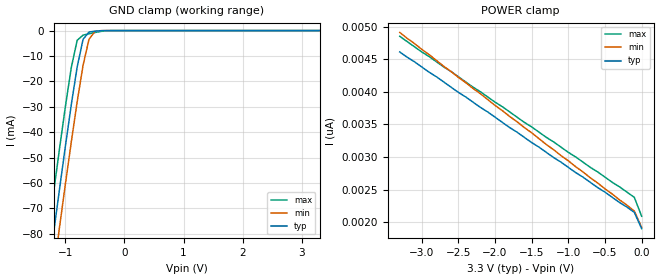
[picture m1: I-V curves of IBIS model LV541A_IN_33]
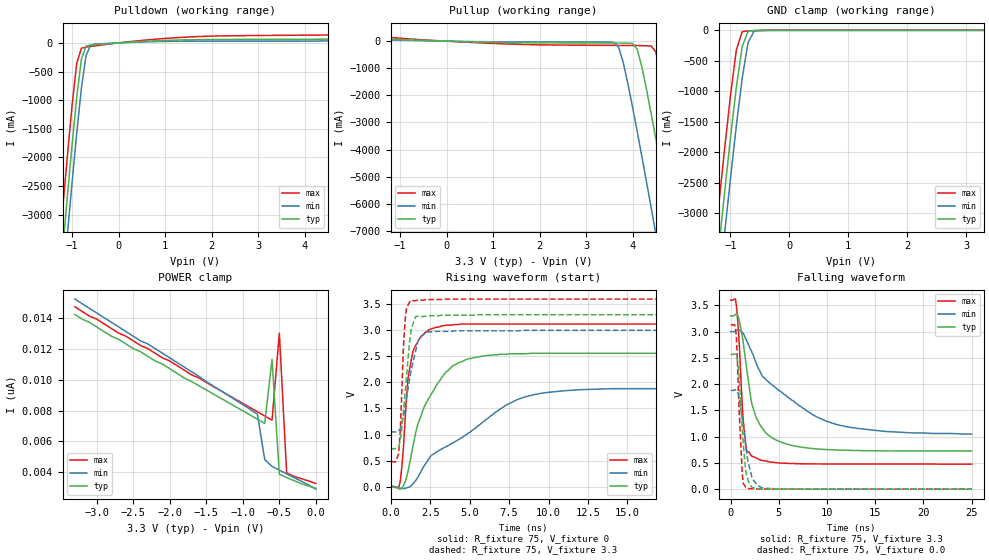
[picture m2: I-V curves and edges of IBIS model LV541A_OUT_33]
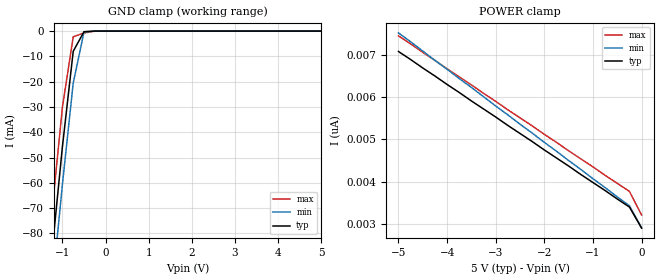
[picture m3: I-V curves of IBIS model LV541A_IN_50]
| TEXAS INSTRUMENTS INCORPORATED
| Standard Linear and Logic Group
| IBIS Model of SN74LV541A
| OCTAL BUFFER/DRIVER WITH 3-STATE OUTPUTS
| SOIC 20-pin (DW), SOP 20-pin (NS), SSOP 20-pin (DB), TSSOP 20-pin (PW)
| and TVSOP 20-pin (DGV) Package
[IBIS Ver]   3.2
[Comment Char]  |_char
[File Name]   lv541a.ibs
[File Rev]   2.0 H_die
[Date]   May 29, 2000
[Source]   Data created from HSPICE simulations at TI-SLL.
[Notes]   The following is an IBIS list for the LV541A.
|   Please contact sllibis@ti.com with questions and
|   comments concerning SLL IBIS models.
|   The warning about non-monotonic V-I curves might be reported,
|   but it is nano ampere region and negligible.
[Disclaimer] Property of Texas Instruments Incorporated.  Unauthorized
   reproduction and/or distribution is strictly prohibited.
   This product is protected under copyright law.
   Created 2000, (C) Copyright 2000, Texas Instruments Inc.,
   All Rights Reserved.
   UNLESS THERE IS A SIGNED, WRITTEN AGREEMENT TO THE
   CONTRARY, TEXAS INSTRUMENTS () IS PROVIDING THE IBIS
   MODELS  AND WITHOUT ANY WARRANTY, EXPRESSED OR
   IMPLIED.  TI assumes no liability for:
   1) the accuracy of the IBIS models provided to your
   company;
   2) the proper functioning of these IBIS Models in your
   design or for any resulting applications; or
   3) infringement of patents, copyrights or intellectual
   property rights resulting from your use of these IBIS
   models.
   TI provides IBIS Models as a service to our customers.
   You and your company shall not distribute, sell or give
   these models to anyone else without prior written
   permission from TI.
   TI reserves the right to make changes to our products or
   to discontinue any semiconductor product or service
   without notice, and advises our customers to obtain the
   latest version of relevant information to verify, before
   placing orders, that the information being relied on is
   current.
   Please be aware that your receipt and use of the IBIS
   information provided shall serve as acceptance of these
   terms and conditions.  If you do not accept these terms,
   you should return or destroy the IBIS models and any
   other accompanying information immediately.
|   Component LV541A_DW
[Component]   LV541A_DW
[Manufacturer]  Texas Instruments, Inc.
[Package]
|   typ   min   max
R_pkg   0.038   0.033   0.045
L_pkg   5.012nH   4.110nH   6.349nH
C_pkg   0.717pF   0.530pF   0.868pF
[Pin]   signal_name   model_name   R_pin   L_pin   C_pin
1   OE1_NOT   LV541A_IN   0.042   6.336nH   0.865pF
2   A1   LV541A_IN   0.043   5.542nH   0.867pF
3   A2   LV541A_IN   0.034   4.714nH   0.732pF
4   A3   LV541A_IN   0.034   4.377nH   0.591pF
5   A4   LV541A_IN   0.036   4.130nH   0.533pF
6   A5   LV541A_IN   0.035   4.111nH   0.530pF
7   A6   LV541A_IN   0.034   4.284nH   0.583pF
8   A7   LV541A_IN   0.034   4.634nH   0.726pF
9   A8   LV541A_IN   0.040   5.518nH   0.865pF
10   GND   GND   0.043   6.349nH   0.866pF
11   Y8   LV541A_OUT   0.041   6.281nH   0.861pF
12   Y7   LV541A_OUT   0.045   5.561nH   0.868pF
13   Y6   LV541A_OUT   0.033   4.778nH   0.742pF
14   Y5   LV541A_OUT   0.035   4.414nH   0.596pF
15   Y4   LV541A_OUT   0.035   4.110nH   0.533pF
16   Y3   LV541A_OUT   0.036   4.130nH   0.533pF
17   Y2   LV541A_OUT   0.034   4.377nH   0.591pF
18   Y1   LV541A_OUT   0.034   4.714nH   0.731pF
19   OE2_NOT   LV541A_IN   0.043   5.569nH   0.868pF
20   VCC   POWER   0.042   6.308nH   0.864pF
|   Component LV541A_NS
[Component]   LV541A_NS
[Manufacturer]  Texas Instruments, Inc.
[Package]
|   typ   min   max
R_pkg   0.044   0.029   0.058
L_pkg   3.666nH   2.317nH   5.115nH
C_pkg   0.548pF   0.316pF   0.725pF
[Pin]   signal_name   model_name   R_pin   L_pin   C_pin
1   OE1_NOT   LV541A_IN   0.058   5.115nH   0.725pF
2   A1   LV541A_IN   0.053   4.591nH   0.724pF
3   A2   LV541A_IN   0.049   3.754nH   0.572pF
4   A3   LV541A_IN   0.029   2.549nH   0.388pF
5   A4   LV541A_IN   0.031   2.317nH   0.316pF
6   A5   LV541A_IN   0.031   2.317nH   0.316pF
7   A6   LV541A_IN   0.029   2.556nH   0.399pF
8   A7   LV541A_IN   0.049   3.754nH   0.579pF
9   A8   LV541A_IN   0.053   4.591nH   0.724pF
10   GND   GND   0.058   5.115nH   0.725pF
11   Y8   LV541A_OUT   0.058   5.115nH   0.725pF
12   Y7   LV541A_OUT   0.053   4.591nH   0.724pF
13   Y6   LV541A_OUT   0.049   3.754nH   0.579pF
14   Y5   LV541A_OUT   0.029   2.557nH   0.399pF
15   Y4   LV541A_OUT   0.031   2.317nH   0.316pF
16   Y3   LV541A_OUT   0.031   2.317nH   0.316pF
17   Y2   LV541A_OUT   0.029   2.557nH   0.399pF
18   Y1   LV541A_OUT   0.049   3.754nH   0.579pF
19   OE2_NOT   LV541A_IN   0.053   4.591nH   0.724pF
20   VCC   POWER   0.058   5.115nH   0.725pF
|   Component LV541A_DB
[Component]   LV541A_DB
[Manufacturer]  Texas Instruments, Inc.
[Package]
|   typ   min   max
R_pkg   0.040   0.035   0.051
L_pkg   3.495nH   3.035nH   4.314nH
C_pkg   0.420pF   0.346pF   0.502pF
[Pin]   signal_name   model_name   R_pin   L_pin   C_pin
1   OE1_NOT   LV541A_IN   0.049   4.310nH   0.502pF
2   A1   LV541A_IN   0.048   3.903nH   0.487pF
3   A2   LV541A_IN   0.035   3.189nH   0.396pF
4   A3   LV541A_IN   0.035   3.036nH   0.347pF
5   A4   LV541A_IN   0.035   3.035nH   0.367pF
6   A5   LV541A_IN   0.035   3.035nH   0.367pF
7   A6   LV541A_IN   0.035   3.036nH   0.347pF
8   A7   LV541A_IN   0.035   3.189nH   0.397pF
9   A8   LV541A_IN   0.047   3.899nH   0.488pF
10   GND   GND   0.051   4.314nH   0.500pF
11   Y8   LV541A_OUT   0.051   4.314nH   0.500pF
12   Y7   LV541A_OUT   0.047   3.899nH   0.488pF
13   Y6   LV541A_OUT   0.035   3.189nH   0.397pF
14   Y5   LV541A_OUT   0.035   3.036nH   0.346pF
15   Y4   LV541A_OUT   0.035   3.035nH   0.367pF
16   Y3   LV541A_OUT   0.035   3.035nH   0.367pF
17   Y2   LV541A_OUT   0.035   3.036nH   0.346pF
18   Y1   LV541A_OUT   0.035   3.189nH   0.397pF
19   OE2_NOT   LV541A_IN   0.047   3.899nH   0.488pF
20   VCC   POWER   0.051   4.314nH   0.502pF
|   Component LV541A_PW
[Component]   LV541A_PW
[Manufacturer]  Texas Instruments, Inc.
[Package]
|   typ   min   max
R_pkg   0.035   0.024   0.047
L_pkg   2.399nH   1.710nH   3.250nH
C_pkg   0.284pF   0.166pF   0.418pF
[Pin]   signal_name   model_name   R_pin   L_pin   C_pin
1   OE1_NOT   LV541A_IN   0.041   3.102nH   0.410pF
2   A1   LV541A_IN   0.040   2.777nH   0.363pF
3   A2   LV541A_IN   0.029   2.194nH   0.260pF
4   A3   LV541A_IN   0.025   1.710nH   0.166pF
5   A4   LV541A_IN   0.025   1.740nH   0.191pF
6   A5   LV541A_IN   0.024   1.763nH   0.193pF
7   A6   LV541A_IN   0.024   1.817nH   0.174pF
8   A7   LV541A_IN   0.028   2.256nH   0.265pF
9   A8   LV541A_IN   0.045   2.887nH   0.368pF
10   GND   GND   0.047   3.250nH   0.417pF
11   Y8   LV541A_OUT   0.046   3.244nH   0.418pF
12   Y7   LV541A_OUT   0.046   2.961nH   0.375pF
13   Y6   LV541A_OUT   0.033   2.334nH   0.268pF
14   Y5   LV541A_OUT   0.029   1.915nH   0.179pF
15   Y4   LV541A_OUT   0.031   1.934nH   0.203pF
16   Y3   LV541A_OUT   0.032   1.917nH   0.201pF
17   Y2   LV541A_OUT   0.030   1.833nH   0.173pF
18   Y1   LV541A_OUT   0.036   2.324nH   0.268pF
19   OE2_NOT   LV541A_IN   0.042   2.869nH   0.372pF
20   VCC   POWER   0.042   3.160nH   0.414pF
|   Component LV541A_DGV
[Component]   LV541A_DGV
[Manufacturer]  Texas Instruments, Inc.
[Package]
|   typ   min   max
R_pkg   0.044   0.038   0.048
L_pkg   2.561nH   2.236nH   2.961nH
C_pkg   0.342pF   0.264pF   0.446pF
[Pin]   signal_name   model_name   R_pin   L_pin   C_pin
1   OE1_NOT   LV541A_IN   0.044   2.935nH   0.417pF
2   A1   LV541A_IN   0.042   2.869nH   0.446pF
3   A2   LV541A_IN   0.043   2.399nH   0.316pF
4   A3   LV541A_IN   0.044   2.236nH   0.265pF
5   A4   LV541A_IN   0.046   2.278nH   0.264pF
6   A5   LV541A_IN   0.045   2.274nH   0.264pF
7   A6   LV541A_IN   0.044   2.285nH   0.269pF
8   A7   LV541A_IN   0.043   2.452nH   0.320pF
9   A8   LV541A_IN   0.044   2.900nH   0.446pF
10   GND   GND   0.044   2.961nH   0.418pF
11   Y8   LV541A_OUT   0.045   2.954nH   0.418pF
12   Y7   LV541A_OUT   0.042   2.847nH   0.443pF
13   Y6   LV541A_OUT   0.045   2.453nH   0.319pF
14   Y5   LV541A_OUT   0.045   2.297nH   0.269pF
15   Y4   LV541A_OUT   0.048   2.334nH   0.268pF
16   Y3   LV541A_OUT   0.048   2.335nH   0.267pF
17   Y2   LV541A_OUT   0.046   2.299nH   0.268pF
18   Y1   LV541A_OUT   0.046   2.457nH   0.320pF
19   OE2_NOT   LV541A_IN   0.043   2.848nH   0.441pF
20   VCC   POWER   0.038   2.812nH   0.408pF
[Model Selector]   LV541A_IN
LV541A_IN_33   3.3-V Vcc Input Model
LV541A_IN_50   5.0-V Vcc Input Model
[Model Selector]   LV541A_OUT
LV541A_OUT_33   3.3-V Vcc Output Model
LV541A_OUT_50   5.0-V Vcc Output Model
| Models and submodels in the file (4): LV541A_IN_33 (Input), LV541A_OUT_33 (3-state), LV541A_IN_50 (Input), LV541A_OUT_50 (3-state)
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|   Model LV541A_IN_33
[Model]   LV541A_IN_33
Model_type  Input
Polarity   Inverting
Vinl = 0.99
Vinh = 2.31
| variable   typ   min   max
C_comp   1.33pf   1.00pf   1.66pf
[Temperature Range]   25   85   -40
[Voltage Range]   3.3   3.0   3.6
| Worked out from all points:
|   GND clamp passes 1 mA (typ) near -0.61 V on its own axis
[GND Clamp]
|   Voltage   I(typ)   I(min)   I(max)
-3.3V     -460mA     -475mA     -445mA
-1.3V     -97.5mA    -113mA     -81.5mA
-1.2V     -79.9mA    -95mA      -63.9mA
-1.1V     -62.6mA    -77.6mA    -46.7mA
-1V       -45.6mA    -60.5mA    -30mA
-900mV    -29.2mA    -43.9mA    -14.6mA
-800mV    -14.3mA    -28mA      -3.81mA
-700mV    -3.42mA    -13.6mA    -1.78mA
-600mV    -581uA     -3.4mA     -1.25mA
-500mV    -233uA     -353uA     -759uA
-400mV    -58.1uA    -21.9uA    -324uA
3.3V      1.9nA      2.34nA     1.69nA
[POWER Clamp]
|   Voltage   I(typ)   I(min)   I(max)
-3.3V     4.61nA     4.91nA     4.85nA
-3V       4.38nA     4.65nA     4.61nA
-100mV    2.15nA     2.17nA     2.38nA
0V        1.9nA      1.92nA     2.09nA
|   Model LV541A_OUT_33
[Model]   LV541A_OUT_33
Model_type  3-state
Polarity   Non-Inverting
Enable   Active-Low
Vinl = 0.99
Vinh = 2.31
Vmeas = 1.65v
Cref = 15pf
| variable   typ   min   max
C_comp   4.60pf   3.45pf   5.75pf
[Temperature Range]   25   85   -40
[Voltage Range]   3.3   3.0   3.6
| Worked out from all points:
|   slope of the pulldown table from 0 to 0.495 V, typ, clamps not added: 19.7 ohm
|   slope of the pullup table from 0 to 0.495 V, typ, clamps not added: 20.4 ohm
|   GND clamp passes 1 mA (typ) near -0.48 V on its own axis
|   rising waveform, R_fixture 75, V_fixture 0: 20-80 % time 1.89ns typ, 4.98ns min, 570ps max; typ from 0 V to 2.56 V
|   falling waveform, R_fixture 75, V_fixture 3.3: 20-80 % time 1.69ns typ, 6.13ns min, 606ps max; typ from 3.3 V to 0.726 V
|   rising waveform, R_fixture 75, V_fixture 3.3: 20-80 % time 456ps typ, 722ps min, 258ps max; typ from 0.726 V to 3.3 V
|   falling waveform, R_fixture 75, V_fixture 0.0: 20-80 % time 570ps typ, 928ps min, 429ps max; typ from 2.57 V to 0 V
[Pulldown]
|   Voltage   I(typ)   I(min)   I(max)
-3.3V     -24.1A     -24.7A     -23.5A
-1.3V     -4.54A     -5.2A      -3.83A
-1.2V     -3.6A      -4.26A     -2.88A
-1.1V     -2.67A     -3.34A     -1.97A
-1V       -1.78A     -2.44A     -1.09A
-900mV    -948mA     -1.58A     -358mA
-800mV    -288mA     -793mA     -92.6mA
-700mV    -55.7mA    -219mA     -74.5mA
-600mV    -37.6mA    -37.4mA    -63.2mA
0V        -3.42nA    -3.55nA    -3.6nA
1.6V      55.7mA     30.4mA     107mA
6.6V      122mA      69mA       228mA
[Pullup]
|   Voltage   I(typ)   I(min)   I(max)
-3.3V     223mA      124mA      415mA
600mV     -28.8mA    -16.4mA    -52.8mA
3.6V      -70.4mA    -45mA      -156mA
3.7V      -71mA      -222mA     -157mA
3.8V      -72.1mA    -794mA     -158mA
4.1V      -302mA     -3.34A     -163mA
4.4V      -2.68A     -6.15A     -177mA
4.5V      -3.6A      -7.11A     -395mA
4.8V      -6.45A     -10A       -2.89A
4.9V      -7.41A     -11A       -3.83A
5.2V      -10.3A     -13.9A     -6.71A
6.6V      -24.1A     -27.7A     -20.5A
[GND Clamp]
|   Voltage   I(typ)   I(min)   I(max)
-3.3V     -24.1A     -24.7A     -23.5A
-1.3V     -4.53A     -5.2A      -3.82A
-1.2V     -3.59A     -4.26A     -2.88A
-1.1V     -2.67A     -3.34A     -1.96A
-1V       -1.77A     -2.44A     -1.08A
-900mV    -938mA     -1.57A     -325mA
-800mV    -266mA     -785mA     -21.9mA
-700mV    -17.6mA    -203mA     -9.17mA
-600mV    -2.58mA    -15.3mA    -6.43mA
-400mV    -298uA     -33.8uA    -1.7mA
3.3V      2.97nA     3.67nA     2.84nA
[POWER Clamp]
|   Voltage   I(typ)   I(min)   I(max)
-3.3V     14.2nA     15.2nA     14.7nA
-2.5V     12nA       12.8nA     12.5nA
-2.4V     11.8nA     12.5nA     12.2nA
-2.3V     11.5nA     12.3nA     12nA
-1.7V     9.87nA     10.5nA     10.3nA
-1.6V     9.6nA      10.2nA     10.1nA
-800mV    7.44nA     7.76nA     7.92nA
-700mV    7.17nA     4.83nA     7.65nA
-600mV    11.3nA     4.39nA     7.38nA
-500mV    3.89nA     4.15nA     13nA
-400mV    3.67nA     3.91nA     3.98nA
0V        2.97nA     2.92nA     3.29nA
[Ramp]
| variable   typ   min   max
dV/dt_r   1.54E+00/1.89E-09   1.14E+00/5.03E-09   1.87E+00/5.53E-10
dV/dt_f   1.57E+00/1.70E-09   1.19E+00/6.17E-09   1.89E+00/5.89E-10
R_load = 75
[Rising Waveform]
R_fixture = 75
V_fixture = 0
|   Time   V(typ)   V(min)   V(max)
0s        0V         0V         0V
600ps     -49.1mV    -28.6mV    89.3mV
800ps     11.1mV     -38.5mV    712mV
1.1ns     292mV      -15mV      2.08V
1.4ns     756mV      52.7mV     2.59V
1.7ns     1.18V      168mV      2.77V
2.4ns     1.69V      524mV      3.01V
4.3ns     2.38V      903mV      3.11V
9ns       2.56V      1.76V      3.12V
25ns      2.56V      1.89V      3.12V
[Falling Waveform]
R_fixture = 75
V_fixture = 3.3
V_fixture_min = 3.0
V_fixture_max = 3.6
|   Time   V(typ)   V(min)   V(max)
0s        3.3V       3V         3.6V
500ps     3.33V      3.01V      3.62V
800ps     3.28V      3.03V      3.04V
1.3ns     2.8V       2.97V      1.32V
1.7ns     2.24V      2.81V      707mV
2.2ns     1.62V      2.61V      629mV
3ns       1.24V      2.26V      563mV
4.1ns     1V         2.01V      516mV
10ns      754mV      1.29V      479mV
25ns      726mV      1.05V      477mV
[Rising Waveform]
R_fixture = 75
V_fixture = 3.3
V_fixture_min = 3.0
V_fixture_max = 3.6
|   Time   V(typ)   V(min)   V(max)
0s        726mV      1.05V      477mV
500ps     766mV      1.06V      627mV
600ps     870mV      1.11V      1.03V
800ps     1.43V      1.34V      2.63V
900ps     1.76V      1.5V       3.14V
1ns       2.11V      1.69V      3.43V
1.3ns     3.01V      2.24V      3.58V
1.8ns     3.27V      2.84V      3.58V
2.3ns     3.28V      2.97V      3.59V
25ns      3.3V       3V         3.6V
[Falling Waveform]
R_fixture = 75
V_fixture = 0.0
|   Time   V(typ)   V(min)   V(max)
0s        2.57V      1.88V      3.13V
500ps     2.57V      1.89V      3.09V
600ps     2.54V      1.88V      2.86V
800ps     2.3V       1.8V       1.88V
1.2ns     1.15V      1.35V      315mV
1.5ns     459mV      919mV      52.1mV
1.7ns     240mV      625mV      14.2mV
2.3ns     30.8mV     187mV      5.9mV
3.3ns     8.02mV     23.2mV     2.94mV
25ns      72.5uV     112uV      75.9uV
|   Model LV541A_IN_50
[Model]   LV541A_IN_50
Model_type  Input
Polarity   Inverting
Vinl = 1.5
Vinh = 3.5
| variable   typ   min   max
C_comp   1.33pf   1.00pf   1.66pf
[Temperature Range]   25   85   -40
[Voltage Range]   5.0   4.5   5.5
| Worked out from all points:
|   GND clamp passes 1 mA (typ) near -0.52 V on its own axis
[GND Clamp]
|   Voltage   I(typ)   I(min)   I(max)
-5V       -773mA     -786mA     -758mA
-1.5V     -133mA     -148mA     -117mA
-1.25V    -88.7mA    -104mA     -72.7mA
-1V       -45.6mA    -60.5mA    -30mA
-750mV    -7.99mA    -20.5mA    -2.23mA
-500mV    -233uA     -353uA     -759uA
-250mV    -2.63nA    -182nA     -26.9uA
5V        2.9nA      3.64nA     2.54nA
[POWER Clamp]
|   Voltage   I(typ)   I(min)   I(max)
-5V       7.08nA     7.52nA     7.45nA
-1.5V     4.37nA     4.5nA      4.73nA
-250mV    3.4nA      3.43nA     3.77nA
0V        2.9nA      2.91nA     3.21nA
